| TI OMAPL137 ZKB IBIS MODEL
[IBIS Ver] 4.1
[File Name]  omapl137b.ibs
[File Rev] 2.0
[Date]  August 6, 2013
[Source] File originated at Texas Instruments.
[Notes]
| (1) First Revision
| (2) Update bc3350bshypbfzp18 model
[Disclaimer] Please be aware that in the absence of a written agreement
| Texas Instruments(TI) assumes no liability for:
| (1) The accuracy of the IBIS models provided to your company
| (2) The proper functioning of these Models in your design
| or for any resulting applications;or
| (3) Infringement of patents,copyrights, or intellectual
| property rights resulting from your use of these models.
| TI provides IBIS Models as a service to our customers and
| therefore reserves the right to limit distribution of the
| Models.
[Copyright] Property of Texas Instruments Incorporated.
| Unauthorized reproduction and/or distribution is strictly
| prohibited.
| This product is protected under copyright law and trade
| secret law as an unpublished work.
| Created 2008,(C) Copyright 2008,
| Texas Instruments Incorporated., All Rights Reserved.
| These commodities are under the U.S.
| Government distribution license control.As such,they are not
| to be re-exported without the prior approval of the U.S.
| Department of Commerce.
| Component OMAPL137_ZKB
[Component]  OMAPL137
[Manufacturer] Texas Instruments
[Package]
| variable  typ   min   max
  R_pkg   3.64204e-001   2.82401e-001   5.04415e-001
  L_pkg   5.31229e-009   3.36760e-009   8.27700e-009
  C_pkg   9.30121e-013   7.13922e-013   1.41974e-012
[Pin] signal_name   model_name   R_pin   L_pin   C_pin
B4   ACLKR0   BC3350BSHYPBFZP18 3.52809e-001 5.60950e-009 8.76837e-013
L2   ACLKR1   BC3350BSHYPBFZP18 3.46358e-001 5.38330e-009 8.26700e-013
C5   ACLKX0   BC3350BSHYPBFZP18 3.66167e-001 4.88250e-009 1.20728e-012
K3   ACLKX1   BC3350BSHYPBFZP18 3.12831e-001 4.27800e-009 9.20188e-013
C4   AFSR0_GP312   BC3350BSHYPBFZP18 3.34079e-001 5.10570e-009 9.86812e-013
L3   AFSR1_GP413   BC3350BSHYPBFZP18 3.12299e-001 4.54110e-009 9.30619e-013
D5   AFSX0   BC3350BSHYPBFZP18 3.71477e-001 5.08500e-009 1.24834e-012
K4   AFSX1   BC3350BSHYPBFZP18 3.41765e-001 4.24400e-009 1.04442e-012
A4   AHCLKR0   BC3350BSHYPBFZP18 3.76725e-001 5.98990e-009 8.52778e-013
L1   AHCLKR1   BC3350BSHYPBFZP18 3.69815e-001 5.86190e-009 7.70130e-013
B5   AHCLKX0   BC3350BSHYPBFZP18 3.58982e-001 5.37680e-009 8.50973e-013
K2   AHCLKX1   BC3350BSHYPBFZP18 3.30094e-001 4.91780e-009 9.16567e-013
L4   AMUTE0   BC3350BSHYPBFZP18 3.09576e-001 3.76710e-009 9.91481e-013
D4   AMUTE1   BC3350BSHYPBFZP18 3.77055e-001 5.45230e-009 1.33440e-012
B8   AXR00   BC3350BSHYPBFZP18 3.42980e-001 4.54010e-009 8.24323e-013
C8   AXR01   BC3350BSHYPBFZP18 3.40691e-001 4.04480e-009 9.24591e-013
D8   AXR02   BC3350BSHYPBFZP18 3.75954e-001 4.33320e-009 9.54888e-013
A7   AXR03   BC3350BSHYPBFZP18 3.64639e-001 5.33620e-009 7.43348e-013
B7   AXR04   BC3350BSHYPBFZP18 3.43602e-001 4.73690e-009 8.47710e-013
C7   AXR05   BC3350BSHYPBFZP18 3.44576e-001 4.05730e-009 9.05082e-013
D7   AXR06   BC3350BSHYPBFZP18 3.69461e-001 4.34900e-009 9.94753e-013
A6   AXR07   BC3350BSHYPBFZP18 3.67219e-001 5.44540e-009 7.46557e-013
B6   AXR08   BC3350BSHYPBFZP18 3.53750e-001 5.03940e-009 8.59768e-013
A5   AXR011   BC3350BSHYPBFZP18 3.73764e-001 5.76780e-009 8.13161e-013
T3   AXR10_GP40   BC3350BSHYPBFZP18 4.02371e-001 6.61940e-009 8.39058e-013
R2   AXR11_GP41   BC3350BSHYPBFZP18 3.58178e-001 5.97780e-009 8.45208e-013
P2   AXR12_GP42   BC3350BSHYPBFZP18 3.42791e-001 5.64970e-009 8.88975e-013
P1   AXR13_EQEP1A_GP43 BC3350BSHYPBFZP18 3.63566e-001 6.03100e-009 9.20426e-013
N2   AXR14_EQEP1B_GP44 BC3350BSHYPBFZP18 3.41482e-001 5.50200e-009 9.27798e-013
N1   AXR15_EPWM2B_GP45 BC3350BSHYPBFZP18 3.65922e-001 6.07060e-009 8.80613e-013
M4   AXR16_EPWM2A_GP46 BC3350BSHYPBFZP18 2.82401e-001 3.36760e-009 9.36204e-013
M3   AXR17_EPWM1B_GP47 BC3350BSHYPBFZP18 3.20269e-001 4.55410e-009 8.47198e-013
M2   AXR18_EPWM1A_GP48 BC3350BSHYPBFZP18 3.43132e-001 5.34010e-009 8.10206e-013
M1   AXR19_GP49   BC3350BSHYPBFZP18 3.70485e-001 5.95560e-009 8.22750e-013
N3   AXR110_GP510   BC3350BSHYPBFZP18 3.94856e-001 5.99760e-009 1.09113e-012
T4   AXR111_GP511   BC3350BSHYPBFZP18 4.03578e-001 6.43790e-009 8.59238e-013
T9   EMAA0_LCDD7_GP10  BC3350BSHYPBFZP18 3.62253e-001 5.18390e-009 7.13922e-013
R9   EMAA1   BC3350BSHYPBFZP18 3.36280e-001 4.65290e-009 7.61440e-013
P9   EMAA2   BC3350BSHYPBFZP18 3.38507e-001 4.20430e-009 9.16635e-013
N9   EMAA3   BC3350BSHYPBFZP18 3.72593e-001 4.70250e-009 1.01617e-012
T10  EMAA4   BC3350BSHYPBFZP18 3.59910e-001 5.10860e-009 7.33343e-013
R10  EMAA5   BC3350BSHYPBFZP18 3.36242e-001 4.69490e-009 7.30442e-013
P10  EMAA6   BC3350BSHYPBFZP18 3.54591e-001 3.81260e-009 9.21521e-013
N10  EMAA7   BC3350BSHYPBFZP18 3.52405e-001 4.07570e-009 8.97300e-013
T11  EMAA8   BC3350BSHYPBFZP18 3.57905e-001 5.25490e-009 7.72078e-013
R11  EMAA9   BC3350BSHYPBFZP18 3.39960e-001 4.95800e-009 7.74933e-013
N8   EMAA10   BC3350BSHYPBFZP18 3.75097e-001 4.22130e-009 9.73411e-013
P11  EMAA11   BC3350BSHYPBFZP18 3.38860e-001 3.99520e-009 9.25534e-013
N11  EMAA12   BC3350BSHYPBFZP18 4.17594e-001 6.33400e-009 1.02745e-012
R8   EMABA0   BC3350BSHYPBFZP18 3.81494e-001 5.55950e-009 8.23734e-013
P8   EMABA1   BC3350BSHYPBFZP18 3.54566e-001 4.27810e-009 9.00141e-013
L16  EMACASn   BC3350BSHYPBFZP18 3.92938e-001 6.23800e-009 8.71406e-013
R12  EMACLK   BC3350BSHYPBFZP18 3.39202e-001 5.16940e-009 7.97026e-013
T8   EMACS0n   BC3350BSHYPBFZP18 3.66291e-001 5.25740e-009 7.51731e-013
P7   EMACS2n   BC3350BSHYPBFZP18 4.03159e-001 5.07700e-009 1.04725e-012
T7   EMACS3n   BC3350BSHYPBFZP18 3.64732e-001 5.37130e-009 7.88748e-013
T13  EMAD0   BC3350BSHYPBFZP18 3.50388e-001 5.52710e-009 7.74650e-013
R15  EMAD1   BC3350BSHYPBFZP18 3.92116e-001 6.67450e-009 1.14113e-012
R13  EMAD2   BC3350BSHYPBFZP18 3.47269e-001 5.79060e-009 1.10354e-012
P15  EMAD3   BC3350BSHYPBFZP18 3.76790e-001 6.19340e-009 9.77386e-013
P13  EMAD4   BC3350BSHYPBFZP18 3.80550e-001 5.98040e-009 1.08166e-012
N15  EMAD5   BC3350BSHYPBFZP18 3.75440e-001 5.94540e-009 1.04784e-012
N13  EMAD6   BC3350BSHYPBFZP18 5.04415e-001 8.27700e-009 1.23154e-012
M15  EMAD7   BC3350BSHYPBFZP18 3.66001e-001 5.73120e-009 9.77509e-013
N12  EMAD8   BC3350BSHYPBFZP18 3.04770e-001 3.65090e-009 1.00494e-012
T14  EMAD9   BC3350BSHYPBFZP18 3.58156e-001 5.85120e-009 8.90599e-013
R14  EMAD10   BC3350BSHYPBFZP18 3.56933e-001 5.78780e-009 1.01396e-012
P16  EMAD11   BC3350BSHYPBFZP18 4.29188e-001 7.33730e-009 1.04270e-012
P14  EMAD12   BC3350BSHYPBFZP18 4.69548e-001 7.98150e-009 1.16936e-012
N16  EMAD13   BC3350BSHYPBFZP18 4.02547e-001 6.61070e-009 9.60829e-013
N14  EMAD14   BC3350BSHYPBFZP18 3.34426e-001 4.96030e-009 1.08614e-012
M16  EMAD15   BC3350BSHYPBFZP18 3.96352e-001 6.45020e-009 9.02472e-013
R7   EMAOEn   BC3350BSHYPBFZP18 3.65530e-001 4.55580e-009 9.39001e-013
N7   EMARASn   BC3350BSHYPBFZP18 3.82760e-001 4.57310e-009 9.92707e-013
T12  EMASDCKE   BC3350BSHYPBFZP18 3.60412e-001 5.45630e-009 7.57754e-013
N6   EMAWAIT0   BC3350BSHYPBFZP18 4.47376e-001 6.98500e-009 1.03580e-012
M13  EMAWEn   BC3350BSHYPBFZP18 3.44034e-001 4.59610e-009 1.06812e-012
M14  EMAWEDQM0n   BC3350BSHYPBFZP18 3.35647e-001 4.86250e-009 1.02092e-012
P12  EMAWEDQM1n   BC3350BSHYPBFZP18 3.66790e-001 4.73480e-009 9.17167e-013
D10  EMBA0_GP72   BC3350BSHYPBFZP18 3.77058e-001 4.39720e-009 9.34609e-013
C10  EMBA1_GP73   BC3350BSHYPBFZP18 3.39593e-001 4.06020e-009 8.73026e-013
B10  EMBA2_GP74   BC3350BSHYPBFZP18 3.40842e-001 4.46430e-009 8.20792e-013
A10  EMBA3_GP75   BC3350BSHYPBFZP18 3.59675e-001 5.14290e-009 7.50346e-013
D11  EMBA4_GP76   BC3350BSHYPBFZP18 4.60149e-001 7.25870e-009 1.10594e-012
C11  EMBA5_GP77   BC3350BSHYPBFZP18 3.56206e-001 4.34760e-009 9.30708e-013
B11  EMBA6_GP78   BC3350BSHYPBFZP18 3.39307e-001 4.75940e-009 8.29396e-013
A11  EMBA7_GP79   BC3350BSHYPBFZP18 3.59232e-001 5.35930e-009 7.70981e-013
D12  EMBA8_GP710   BC3350BSHYPBFZP18 4.50924e-001 6.39680e-009 1.16313e-012
C12  EMBA9_GP711   BC3350BSHYPBFZP18 3.50976e-001 4.60980e-009 1.00328e-012
A9   EMBA10_GP712   BC3350BSHYPBFZP18 3.62039e-001 5.23120e-009 7.40841e-013
B12  EMBA11_GP713   BC3350BSHYPBFZP18 3.37383e-001 4.87380e-009 8.11411e-013
B15  EMBA12_GP313   BC3350BSHYPBFZP18 3.85664e-001 6.59770e-009 9.14478e-013
C9   EMBBA0_GP71   BC3350BSHYPBFZP18 3.40826e-001 4.11030e-009 8.91571e-013
B9   EMBBA1_GP70   BC3350BSHYPBFZP18 3.41753e-001 4.77660e-009 7.89530e-013
L13  EMBCASn   BC3350BSHYPBFZP18 3.42814e-001 4.23070e-009 1.09552e-012
C14  EMBCLK   BC3350BSHYPBFZP18 3.09496e-001 4.71760e-009 1.00435e-012
D9   EMBCS0n   BC3350BSHYPBFZP18 3.82529e-001 4.18540e-009 1.02527e-012
F16  EMBD0_GP60   BC3350BSHYPBFZP18 3.81418e-001 6.10250e-009 8.54913e-013
G13  EMBD1_GP61   BC3350BSHYPBFZP18 3.16694e-001 3.87050e-009 9.12777e-013
G16  EMBD2_GP62   BC3350BSHYPBFZP18 3.74841e-001 5.89880e-009 8.18098e-013
H13  EMBD3_GP63   BC3350BSHYPBFZP18 3.23785e-001 3.89390e-009 9.62755e-013
H16  EMBD4_GP64   BC3350BSHYPBFZP18 3.79284e-001 5.84310e-009 7.97857e-013
J13  EMBD5_GP65   BC3350BSHYPBFZP18 3.28927e-001 3.90710e-009 9.61338e-013
J15  EMBD6_GP66   BC3350BSHYPBFZP18 3.56737e-001 5.35660e-009 7.99572e-013
J16  EMBD7_GP67   BC3350BSHYPBFZP18 3.77816e-001 5.84460e-009 7.43550e-013
C16  EMBD8_GP68   BC3350BSHYPBFZP18 3.80933e-001 6.47220e-009 8.27697e-013
D13  EMBD9_GP69   BC3350BSHYPBFZP18 3.45233e-001 5.24100e-009 1.06722e-012
D14  EMBD10_GP610   BC3350BSHYPBFZP18 3.84203e-001 5.96840e-009 1.18593e-012
D15  EMBD11_GP611   BC3350BSHYPBFZP18 3.74175e-001 6.11540e-009 1.03615e-012
D16  EMBD12_GP612   BC3350BSHYPBFZP18 3.78250e-001 6.27890e-009 8.84231e-013
E13  EMBD13_GP613   BC3350BSHYPBFZP18 3.12049e-001 3.78950e-009 9.79355e-013
E16  EMBD14_GP614   BC3350BSHYPBFZP18 3.76442e-001 6.02250e-009 7.95484e-013
F13  EMBD15_GP615   BC3350BSHYPBFZP18 3.08365e-001 3.74670e-009 8.89905e-013
G15  EMBD16   BC3350BSHYPBFZP18 3.58821e-001 5.47240e-009 8.24972e-013
H14  EMBD17   BC3350BSHYPBFZP18 3.26735e-001 4.48970e-009 9.41389e-013
H15  EMBD18   BC3350BSHYPBFZP18 3.58195e-001 5.28430e-009 8.19685e-013
J14  EMBD19   BC3350BSHYPBFZP18 3.28117e-001 4.37670e-009 9.04122e-013
K13  EMBD20   BC3350BSHYPBFZP18 3.29721e-001 4.04190e-009 8.89989e-013
K16  EMBD21   BC3350BSHYPBFZP18 3.88893e-001 6.11000e-009 8.98496e-013
L14  EMBD22   BC3350BSHYPBFZP18 3.32673e-001 4.65120e-009 1.00366e-012
L15  EMBD23   BC3350BSHYPBFZP18 3.63068e-001 5.54920e-009 9.09082e-013
A13  EMBD24   BC3350BSHYPBFZP18 3.69123e-001 5.90040e-009 7.59127e-013
B14  EMBD25   BC3350BSHYPBFZP18 3.71273e-001 6.13490e-009 8.96553e-013
A14  EMBD26   BC3350BSHYPBFZP18 3.95925e-001 6.62640e-009 9.20786e-013
E14  EMBD27   BC3350BSHYPBFZP18 3.19926e-001 4.62610e-009 8.99241e-013
E15  EMBD28   BC3350BSHYPBFZP18 3.52886e-001 5.56830e-009 8.79877e-013
F14  EMBD29   BC3350BSHYPBFZP18 3.12588e-001 4.41710e-009 9.01046e-013
F15  EMBD30   BC3350BSHYPBFZP18 3.59556e-001 5.57550e-009 8.85265e-013
G14  EMBD31   BC3350BSHYPBFZP18 4.47414e-001 6.82670e-009 1.06701e-012
A8   EMBRASn   BC3350BSHYPBFZP18 3.63563e-001 5.14060e-009 7.63955e-013
C13  EMBSDCKE   BC3350BSHYPBFZP18 3.10671e-001 4.63030e-009 9.43484e-013
K15  EMBWEn   BC3350BSHYPBFZP18 3.59279e-001 5.40410e-009 8.86802e-013
K14  EMBWEDQM0n_GP515  BC3350BSHYPBFZP18 3.25276e-001 4.42660e-009 9.41279e-013
C15  EMBWEDQM1n_GP514  BC3350BSHYPBFZP18 3.30920e-001 5.48860e-009 8.27015e-013
B13  EMBWEDQM2n   BC3350BSHYPBFZP18 3.48317e-001 5.25540e-009 8.14938e-013
A12  EMBWEDQM3n   BC3350BSHYPBFZP18 3.62486e-001 5.39860e-009 7.43677e-013
J5   EMU0_GP715   BC3350BSHYPBFZP18 3.69046e-001 4.50990e-009 1.16280e-012
|F2  OSCIN   IQOSC0002   3.70309e-001 5.68730e-009 9.35563e-013
G3   RESETN   IHHV33SP18   3.44171e-001 4.95330e-009 9.13499e-013
|H1  RTC_XI   IQOSC0002   3.63277e-001 5.85200e-009 8.77945e-013
K1   RTCK_GP714   BC3350BSHYPBFZP18 3.77799e-001 5.82520e-009 7.55951e-013
T5   SPI0CLK   BC3350BSHYPBFZP18 3.97676e-001 6.09390e-009 8.53664e-013
R5   SPI0ENAn   BC3350BSHYPBFZP18 3.71665e-001 5.87670e-009 9.14121e-013
N4   SPI0SCS0n   BC3350BSHYPBFZP18 4.20016e-001 6.21340e-009 1.41974e-012
P6   SPI0SIMO0   BC3350BSHYPBFZP18 4.39152e-001 7.00930e-009 1.01319e-012
R6   SPI0SOMI0   BC3350BSHYPBFZP18 4.10743e-001 6.49310e-009 9.44051e-013
T6   SPI1CLK   BC3350BSHYPBFZP18 3.72427e-001 5.54970e-009 8.18960e-013
N5   SPI1SIMO0   BC3350BSHYPBFZP18 4.30795e-001 6.01870e-009 1.23831e-012
P5   SPI1SOMI0   BC3350BSHYPBFZP18 4.11569e-001 5.82620e-009 1.20256e-012
H3   TCK   BC3350BSHYPBFZP18 3.60260e-001 4.74040e-009 1.07627e-012
J2   TDI   BC3350BSHYPBFZP18 3.23366e-001 4.54700e-009 8.62630e-013
J3   TDO   BC3350BSHYPBFZP18 4.05022e-001 6.03360e-009 9.97296e-013
J1   TMS   BC3350BSHYPBFZP18 3.78273e-001 5.80060e-009 8.59512e-013
J4   TRSTN   BC3350BSHYPBFZP18 3.34544e-001 3.99940e-009 8.85790e-013
R3   UART0RXD   BC3350BSHYPBFZP18 3.53771e-001 5.81880e-009 9.73858e-013
P3   UART0TXD   BC3350BSHYPBFZP18 4.38117e-001 7.34150e-009 1.05073e-012
C6   UART1RXD   BC3350BSHYPBFZP18 3.57344e-001 4.22800e-009 9.58743e-013
D6   UART1TXD   BC3350BSHYPBFZP18 3.80836e-001 4.82410e-009 1.29126e-012
R4   SPI1ENAn   BC3350BSHYPBFZP18 3.77550e-001 6.07530e-009 9.00732e-013
P4   SPI1SCS0n   BC3350BSHYPBFZP18 4.08458e-001 6.42790e-009 1.00073e-012
E4   USB0DRVVBUS   BC3350BSHYPBFZP18 3.71854e-001 5.95540e-009 1.22560e-012
G4   USB0_DM   USB_DATA_DM   2.16E-01   3.52E-09   5.17E-13
F4   USB0_DP   USB_DATA_DP   2.15E-01   3.53E-09   5.99E-13
F7   RESERVED   NC
B1   RESERVED   NC
F3   NC   NC
H4   NC   NC
F6   CVDD   POWER
G6   CVDD   POWER
G7   CVDD   POWER
G10  CVDD   POWER
G11  CVDD   POWER
H7   CVDD   POWER
H10  CVDD   POWER
H11  CVDD   POWER
J6   CVDD   POWER
J7   CVDD   POWER
J10  CVDD   POWER
J11  CVDD   POWER
J12  CVDD   POWER
K6   CVDD   POWER
K7   CVDD   POWER
K10  CVDD   POWER
K11  CVDD   POWER
L6   CVDD   POWER
H6   RVDD   POWER
H12  RVDD   POWER
B16  DVDD   POWER
E5   DVDD   POWER
E8   DVDD   POWER
E9   DVDD   POWER
E12  DVDD   POWER
F5   DVDD   POWER
F11  DVDD   POWER
F12  DVDD   POWER
G5   DVDD   POWER
G12  DVDD   POWER
K5   DVDD   POWER
K12  DVDD   POWER
L5   DVDD   POWER
L11  DVDD   POWER
L12  DVDD   POWER
M5   DVDD   POWER
M8   DVDD   POWER
M9   DVDD   POWER
M12  DVDD   POWER
R1   DVDD   POWER
R16  DVDD   POWER
A1   VSS   GND
A2   VSS   GND
A15  VSS   GND
A16  VSS   GND
B2   VSS   GND
E6   VSS   GND
E7   VSS   GND
E10  VSS   GND
E11  VSS   GND
F8   VSS   GND
F9   VSS   GND
F10  VSS   GND
G8   VSS   GND
G9   VSS   GND
H8   VSS   GND
H9   VSS   GND
J8   VSS   GND
J9   VSS   GND
K8   VSS   GND
K9   VSS   GND
L7   VSS   GND
L8   VSS   GND
L9   VSS   GND
L10  VSS   GND
M6   VSS   GND
M7   VSS   GND
M10  VSS   GND
M11  VSS   GND
T1   VSS   GND
T2   VSS   GND
T15  VSS   GND
T16  VSS   GND
E2   OSCVSS   GND
D1   PLL0_VDDA   POWER
E1   PLL0_VSSA   GND
G2   RTC_VSS   GND
H5   USB0_VDDA33   POWER
E3   USB0_VDDA18   POWER
C3   USB0_VDDA12   POWER
D2   USB0_ID   NC
D3   USB0_VBUS   POWER
[Model Selector] BC3350BSHYPBFZP18
WK_PD_ON_3P3  Cell operated at 3.3(nom)
|WK_PD_ON_3P3; WEAK_PULLDOWN_ON
WK_PU_ON_3P3  Cell operated at 3.3(nom)
|WK_PU_ON_3P3; WEAK_PULLUP_ON
DRIVER_MODE_3P3  Cell operated at 3.3(nom)
|DRIVER_MODE_3P3
[Model Selector] USB_DATA_DP
hs_dp   usb dp for high speed mode
fs_dp   usb dp for full speed mode
[Model Selector] USB_DATA_DM
hs_dm   usb dm for high speed mode
fs_dm   usb dm for full speed mode
| Models and submodels in the file (8): IHHV33SP18 (Input), WK_PD_ON_3P3 (Input), WK_PU_ON_3P3 (Input), DRIVER_MODE_3P3 (I/O), hs_dp (3-state), hs_dm (3-state), fs_dp (3-state), fs_dm (3-state)
